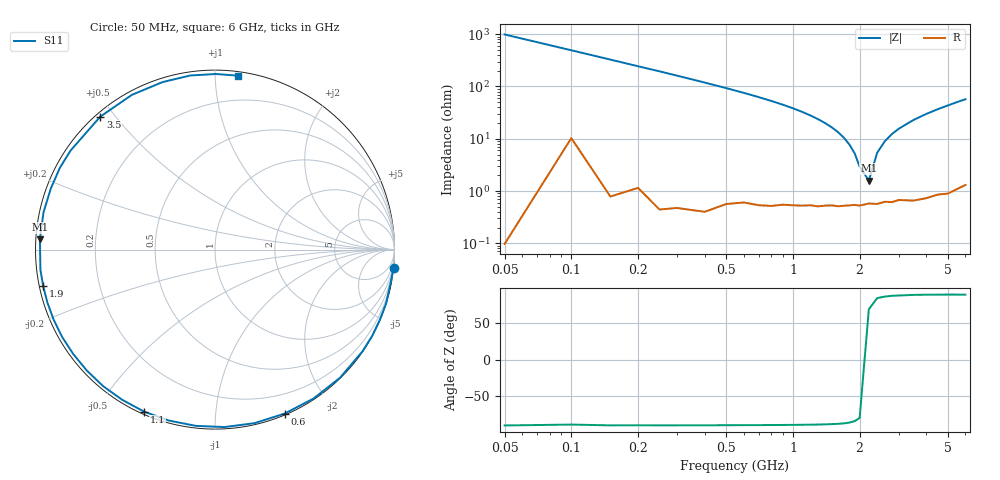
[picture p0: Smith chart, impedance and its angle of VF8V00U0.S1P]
! Infineon Technologies  Discrete & RF Semiconductors
! BBY 58-03
! Si Tuning Diode in SOD323
! VR = 8 V
! S-Parameters:  June  1999
# GHz  S  MA  R  50
!  f  S11
! GHz  MAG  ANG
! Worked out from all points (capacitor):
!   34 points, 50 MHz to 6 GHz, reference 50 ohm
!   read as one part to ground: C = 3.23 pF near 50 MHz
!   lowest |Z| = 1.59 ohm at 2.2 GHz (marker M1)
!   series resonance near 2.132 GHz, so ESL is about 1.7 nH
!   S11 on the Smith chart (normalised r, x): 50 MHz: 0, -20; 600 MHz: 0.01, -1.51; 1.1 GHz: 0.01, -0.65; 1.9 GHz: 0.01, -0.10; 3.5 GHz: 0.01, +0.46; 6 GHz: 0.03, +1.14
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0.05  1 -5.8
0.15  0.9993 -17.4
0.25  0.9989 -28.8
0.3  0.9983 -34.5
0.4  0.9976 -45.7
0.5  0.9949 -56.5
0.6  0.9927 -67.0
0.7  0.9917 -77.2
0.8  0.9902 -86.9
0.9  0.9879 -96.2
1  0.9866 -105.1
1.1  0.9854 -113.6
1.3  0.9835 -129.4
1.4  0.9819 -136.7
1.6  0.981 -150.2
1.7  0.9801 -156.5
1.9  0.9787 -168.1
2  0.9792 -173.4
2.2  0.9771 176.6
2.4  0.9778 167.7
2.8  0.977 152.2
3  0.9756 145.5
3.5  0.9785 130.8
4  0.9786 118.2
4.5  0.978 107.4
5  0.9798 98.1
5.5  0.9785 89.7
6  0.9775 82.5
